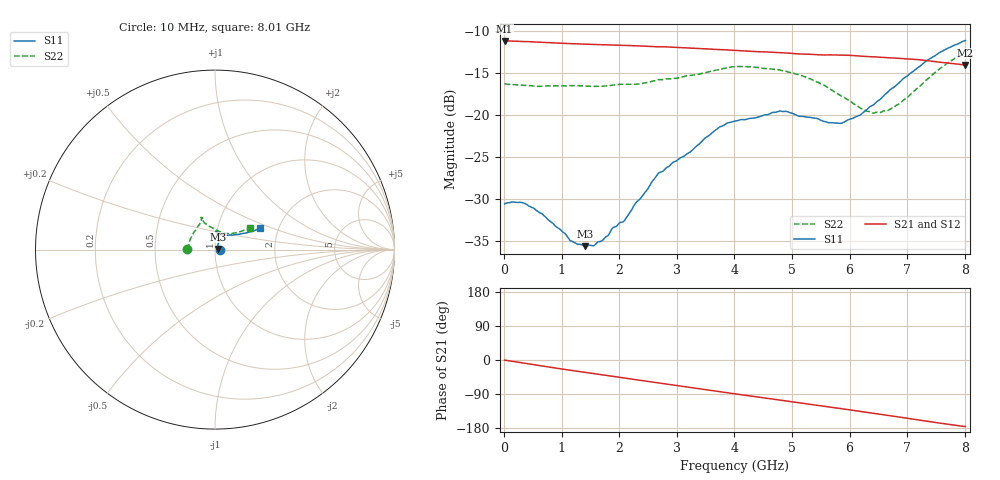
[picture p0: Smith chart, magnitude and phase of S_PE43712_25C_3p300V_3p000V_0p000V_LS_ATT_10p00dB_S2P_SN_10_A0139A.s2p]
! DEVICE ID: PE43712
! File Path: z:\PE43713\PE43713_CHAR_NOM_04292014\AMB\3p300\LS_ATT_10p00dB\PE43713_AMB_3p300V_3p000V_0p000V_LS_ATT_10p00dB_S2P_SN_10_A0139A.s2p
! Serial: 10
! Lot: A0139A
! Temp: 25C
! VDD: 3.300
! VSS: 0.000
! Control_Hi: 3.000
! Control_Lo: 0.000
! Attenuation Step: 10.00dB
! Port 1: RF1
! Port 2: RF2
! ThroughPath:1-2
! IDD: 0.0001466616
! ISS: -6.97e-008
#  Hz  S  RI  R  50
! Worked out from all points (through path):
!   801 points, 10 MHz to 8.01 GHz, reference 50 ohm
!   highest |S21| = -11.17 dB at 10 MHz (marker M1); lowest = -14.0 dB at 8 GHz (marker M2)
!   group delay of S21, straight-line fit = 60.3 ps
!   lowest |S11| = -35.6 dB at 1.41 GHz (marker M3), VSWR 1.03, Z = 51.7 + j0.369 ohm
!   |S11| at or under -10 dB: start of sweep to end of sweep
!   |S22| runs from -19.8 to -12.8 dB; largest |S21 - S12| = 0.001
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1e7  0.0297 0.000141  0.2764 -0.00151  0.2766 -0.00139  -0.1537 0.00101
3.7e8  0.0296 -0.00346  0.2705 -0.0431  0.2714 -0.0434  -0.1495 0.0181
6.8e8  0.0252 -0.00386  0.26 -0.0766  0.2601 -0.0767  -0.1449 0.0338
1.17e9  0.0179 0.000519  0.2363 -0.1225  0.2363 -0.1227  -0.1388 0.0565
1.35e9  0.0168 0.00265  0.2263 -0.1378  0.2263 -0.1379  -0.135 0.0638
1.41e9  0.0163 0.00357  0.2227 -0.1427  0.2227 -0.1428  -0.1331 0.0669
1.7e9  0.0151 0.00967  0.204 -0.1651  0.204 -0.1651  -0.125 0.0807
2.09e9  0.0146 0.0185  0.1755 -0.1917  0.1756 -0.1916  -0.1161 0.0993
2.68e9  0.0203 0.0404  0.1261 -0.2216  0.126 -0.2217  -0.0928 0.1334
3.24e9  0.017 0.0583  0.0744 -0.2393  0.0744 -0.2393  -0.0807 0.1523
3.72e9  0.0152 0.0826  0.0296 -0.2439  0.0294 -0.2439  -0.0753 0.1707
4.01e9  0.0121 0.0916  0.00277 -0.2429  0.00274 -0.2429  -0.0773 0.1785
4.79e9  0.00706 0.1057  -0.0644 -0.2265  -0.0644 -0.2267  -0.0717 0.1711
5.35e9  0.017 0.095  -0.1061 -0.2039  -0.1061 -0.2038  -0.0607 0.1509
5.88e9  0.0391 0.0813  -0.1425 -0.1774  -0.1422 -0.1774  -0.0251 0.1267
6.18e9  0.0604 0.0799  -0.1601 -0.1574  -0.1597 -0.1575  0.00323 0.1102
6.38e9  0.0793 0.0815  -0.1698 -0.1436  -0.1695 -0.1436  0.0236 0.101
6.68e9  0.112 0.0828  -0.1829 -0.1212  -0.1826 -0.1212  0.0577 0.0907
7.35e9  0.1882 0.0975  -0.2002 -0.0658  -0.2 -0.0658  0.1312 0.0979
7.72e9  0.2268 0.1086  -0.2007 -0.036  -0.2007 -0.0362  0.1731 0.1128
8e9  0.2499 0.1199  -0.198 -0.0158  -0.1977 -0.0161  0.1938 0.1224
8.01e9  0.2506 0.1206  -0.198 -0.0153  -0.1977 -0.0156  0.1944 0.1226
